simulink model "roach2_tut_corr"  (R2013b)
settings: Solver=VariableStepDiscrete  SolverMode=SingleTasking  StartTime=0.0  StopTime=100  RelTol=1e-3
undefined symbols (not defined in the file): add_latency, addr_width, Bit, bitfield, BitWidth, bram_latency, burst_size, casper_library_scopes, conv_latency, data_width, DelayLen, fan_latency, FFTSize, FFTStage, getfield, increment, led, Location, Lower, mult_latency, mux_latency, n_bits, n_bits_data, n_inputs, n_streams, n_taps, neg_latency, negate_latency, nsamples, pfb_size, pulse_len, reset_period, ROACH, ROACH2, snapshot, sx475t, sync_period, sync_period_bits, Upper, UseCounter, Width
libraries: xbsIndex_r4 x24444, casper_library_misc x73, xbsReplacements_r4 x34, casper_library_delays x14, xps_library x7
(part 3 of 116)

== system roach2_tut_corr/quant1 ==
  sync : Inport
  din : Inport  Port=2
  Constant : xbsIndex_r4/Constant  const=0  gui_display_data_type=Fixed-point  arith_type=Unsigned  n_bits=32  bin_pt=0  preci_type=Single  exp_width=8  frac_width=24  explicit_period=on  period=1  equ=P=C  opselect=C  inp2=PCIN>>17  opr=+  inp1=P  carry=CIN  dbl_ovrd=off  block_type=constant
  Constant1 : xbsIndex_r4/Constant  const=0  gui_display_data_type=Boolean  arith_type=Boolean  n_bits=32  bin_pt=0  preci_type=Single  exp_width=8  frac_width=24  explicit_period=on  period=1  equ=P=C  opselect=C  inp2=PCIN>>17  opr=+  inp1=P  carry=CIN  dbl_ovrd=off  block_type=constant
  Counter : xbsIndex_r4/Counter  cnt_type=Free Running  cnt_to=Inf  operation=Up  start_count=0  cnt_by_val=1  arith_type=Unsigned  n_bits=10  bin_pt=0  load_pin=off  rst=on  en=off  explicit_period=on  period=1  dbl_ovrd=off  use_behavioral_HDL=off  implementation=Fabric  block_type=counter
  Delay{1..3,5} (4 alike) : xbsIndex_r4/Delay  rst=off  infoeditControl=Selection of Reset will increase slice count due to use of real FFs and instead of SRLs  en=off  latency=1  dbl_ovrd=off  reg_retiming=on  block_type=delay
  Delay{6,18..19,25} (4 alike) : xbsIndex_r4/Delay  rst=off  infoeditControl=Selection of Reset will increase slice count due to use of real FFs and instead of SRLs  en=off  latency=1  dbl_ovrd=off  reg_retiming=off  block_type=delay
  Delay4 : xbsIndex_r4/Delay  rst=off  infoeditControl=Selection of Reset will increase slice count due to use of real FFs and instead of SRLs  en=off  latency=6  dbl_ovrd=off  reg_retiming=on  block_type=delay
  Logical5 : xbsIndex_r4/Logical  logical_function=OR  inputs=2  en=off  latency=0  precision=Full  arith_type=Unsigned  n_bits=8  bin_pt=2  align_bp=on  dbl_ovrd=off  block_type=logical
  Slice11 : xbsIndex_r4/Slice  nbits=16  boolean_output=off  mode=Lower Bit Location + Width  bit1=0  base1=MSB of Input  bit0=0  base0=LSB of Input  dbl_ovrd=off  block_type=slice
  Slice14 : xbsIndex_r4/Slice  nbits=16  boolean_output=off  mode=Lower Bit Location + Width  bit1=0  base1=MSB of Input  bit0=16  base0=LSB of Input  dbl_ovrd=off  block_type=slice
  bus_expand : Subsystem  AncestorBlock=casper_library_flow_control/bus_expand
  coeffs : Subsystem  Tag=xps:bram  AncestorBlock=xps_library/Shared_BRAM
  round0 : Subsystem
  round1 : Subsystem
  sync_out : Outport
  clip_out : Outport  Port=2
  dout0 : Outport  Port=3
  dout1 : Outport  Port=4
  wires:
  round0/2(clip) -> Logical5/1
  round1/2(clip) -> Logical5/2
  Delay19/1 -> Delay4/1
  coeffs/1(data_out) -> Delay1/1
  Slice14/1 -> round0/2(scale)
  Slice11/1 -> round1/2(scale)
  Delay18/1 -> Delay3/1
  Delay25/1 -> Delay2/1
  sync/1 -> Counter/1, Delay6/1
  Delay4/1 -> sync_out/1
  round0/1(dout) -> dout0/1
  Logical5/1 -> Delay5/1
  bus_expand/2(lsb_out1) -> Delay25/1
  round1/1(dout) -> dout1/1
  Delay1/1 -> Slice11/1, Slice14/1
  Delay2/1 -> round1/1(din)
  Delay3/1 -> round0/1(din)
  Delay5/1 -> clip_out/1
  bus_expand/1(msb_out2) -> Delay18/1
  din/1 -> bus_expand/1(bus_in)
  Delay6/1 -> Delay19/1
  Counter/1 -> coeffs/1(addr)
  Constant/1 -> coeffs/2(data_in)
  Constant1/1 -> coeffs/3(we)

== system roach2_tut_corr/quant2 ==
  sync : Inport
  din : Inport  Port=2
  Constant : xbsIndex_r4/Constant  const=0  gui_display_data_type=Fixed-point  arith_type=Unsigned  n_bits=32  bin_pt=0  preci_type=Single  exp_width=8  frac_width=24  explicit_period=on  period=1  equ=P=C  opselect=C  inp2=PCIN>>17  opr=+  inp1=P  carry=CIN  dbl_ovrd=off  block_type=constant
  Constant1 : xbsIndex_r4/Constant  const=0  gui_display_data_type=Boolean  arith_type=Boolean  n_bits=32  bin_pt=0  preci_type=Single  exp_width=8  frac_width=24  explicit_period=on  period=1  equ=P=C  opselect=C  inp2=PCIN>>17  opr=+  inp1=P  carry=CIN  dbl_ovrd=off  block_type=constant
  Counter : xbsIndex_r4/Counter  cnt_type=Free Running  cnt_to=Inf  operation=Up  start_count=0  cnt_by_val=1  arith_type=Unsigned  n_bits=10  bin_pt=0  load_pin=off  rst=on  en=off  explicit_period=on  period=1  dbl_ovrd=off  use_behavioral_HDL=off  implementation=Fabric  block_type=counter
  Delay{1..3,5} (4 alike) : xbsIndex_r4/Delay  rst=off  infoeditControl=Selection of Reset will increase slice count due to use of real FFs and instead of SRLs  en=off  latency=1  dbl_ovrd=off  reg_retiming=on  block_type=delay
  Delay{6,18..19,25} (4 alike) : xbsIndex_r4/Delay  rst=off  infoeditControl=Selection of Reset will increase slice count due to use of real FFs and instead of SRLs  en=off  latency=1  dbl_ovrd=off  reg_retiming=off  block_type=delay
  Delay4 : xbsIndex_r4/Delay  rst=off  infoeditControl=Selection of Reset will increase slice count due to use of real FFs and instead of SRLs  en=off  latency=6  dbl_ovrd=off  reg_retiming=on  block_type=delay
  Logical5 : xbsIndex_r4/Logical  logical_function=OR  inputs=2  en=off  latency=0  precision=Full  arith_type=Unsigned  n_bits=8  bin_pt=2  align_bp=on  dbl_ovrd=off  block_type=logical
  Slice11 : xbsIndex_r4/Slice  nbits=16  boolean_output=off  mode=Lower Bit Location + Width  bit1=0  base1=MSB of Input  bit0=0  base0=LSB of Input  dbl_ovrd=off  block_type=slice
  Slice14 : xbsIndex_r4/Slice  nbits=16  boolean_output=off  mode=Lower Bit Location + Width  bit1=0  base1=MSB of Input  bit0=16  base0=LSB of Input  dbl_ovrd=off  block_type=slice
  bus_expand : Subsystem  AncestorBlock=casper_library_flow_control/bus_expand
  coeffs : Subsystem  Tag=xps:bram  AncestorBlock=xps_library/Shared_BRAM
  round0 : Subsystem
  round1 : Subsystem
  sync_out : Outport
  clip_out : Outport  Port=2
  dout0 : Outport  Port=3
  dout1 : Outport  Port=4
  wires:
  round0/2(clip) -> Logical5/1
  round1/2(clip) -> Logical5/2
  Delay19/1 -> Delay4/1
  coeffs/1(data_out) -> Delay1/1
  Slice14/1 -> round0/2(scale)
  Slice11/1 -> round1/2(scale)
  Delay18/1 -> Delay3/1
  Delay25/1 -> Delay2/1
  sync/1 -> Counter/1, Delay6/1
  Delay4/1 -> sync_out/1
  round0/1(dout) -> dout0/1
  Logical5/1 -> Delay5/1
  bus_expand/2(lsb_out1) -> Delay25/1
  round1/1(dout) -> dout1/1
  Delay1/1 -> Slice11/1, Slice14/1
  Delay2/1 -> round1/1(din)
  Delay3/1 -> round0/1(din)
  Delay5/1 -> clip_out/1
  bus_expand/1(msb_out2) -> Delay18/1
  din/1 -> bus_expand/1(bus_in)
  Delay6/1 -> Delay19/1
  Counter/1 -> coeffs/1(addr)
  Constant/1 -> coeffs/2(data_in)
  Constant1/1 -> coeffs/3(we)

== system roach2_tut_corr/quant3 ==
  sync : Inport
  din : Inport  Port=2
  Constant : xbsIndex_r4/Constant  const=0  gui_display_data_type=Fixed-point  arith_type=Unsigned  n_bits=32  bin_pt=0  preci_type=Single  exp_width=8  frac_width=24  explicit_period=on  period=1  equ=P=C  opselect=C  inp2=PCIN>>17  opr=+  inp1=P  carry=CIN  dbl_ovrd=off  block_type=constant
  Constant1 : xbsIndex_r4/Constant  const=0  gui_display_data_type=Boolean  arith_type=Boolean  n_bits=32  bin_pt=0  preci_type=Single  exp_width=8  frac_width=24  explicit_period=on  period=1  equ=P=C  opselect=C  inp2=PCIN>>17  opr=+  inp1=P  carry=CIN  dbl_ovrd=off  block_type=constant
  Counter : xbsIndex_r4/Counter  cnt_type=Free Running  cnt_to=Inf  operation=Up  start_count=0  cnt_by_val=1  arith_type=Unsigned  n_bits=10  bin_pt=0  load_pin=off  rst=on  en=off  explicit_period=on  period=1  dbl_ovrd=off  use_behavioral_HDL=off  implementation=Fabric  block_type=counter
  Delay{1..3,5} (4 alike) : xbsIndex_r4/Delay  rst=off  infoeditControl=Selection of Reset will increase slice count due to use of real FFs and instead of SRLs  en=off  latency=1  dbl_ovrd=off  reg_retiming=on  block_type=delay
  Delay{6,18..19,25} (4 alike) : xbsIndex_r4/Delay  rst=off  infoeditControl=Selection of Reset will increase slice count due to use of real FFs and instead of SRLs  en=off  latency=1  dbl_ovrd=off  reg_retiming=off  block_type=delay
  Delay4 : xbsIndex_r4/Delay  rst=off  infoeditControl=Selection of Reset will increase slice count due to use of real FFs and instead of SRLs  en=off  latency=6  dbl_ovrd=off  reg_retiming=on  block_type=delay
  Logical5 : xbsIndex_r4/Logical  logical_function=OR  inputs=2  en=off  latency=0  precision=Full  arith_type=Unsigned  n_bits=8  bin_pt=2  align_bp=on  dbl_ovrd=off  block_type=logical
  Slice11 : xbsIndex_r4/Slice  nbits=16  boolean_output=off  mode=Lower Bit Location + Width  bit1=0  base1=MSB of Input  bit0=0  base0=LSB of Input  dbl_ovrd=off  block_type=slice
  Slice14 : xbsIndex_r4/Slice  nbits=16  boolean_output=off  mode=Lower Bit Location + Width  bit1=0  base1=MSB of Input  bit0=16  base0=LSB of Input  dbl_ovrd=off  block_type=slice
  bus_expand : Subsystem  AncestorBlock=casper_library_flow_control/bus_expand
  coeffs : Subsystem  Tag=xps:bram  AncestorBlock=xps_library/Shared_BRAM
  round0 : Subsystem
  round1 : Subsystem
  sync_out : Outport
  clip_out : Outport  Port=2
  dout0 : Outport  Port=3
  dout1 : Outport  Port=4
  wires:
  round0/2(clip) -> Logical5/1
  round1/2(clip) -> Logical5/2
  Delay19/1 -> Delay4/1
  coeffs/1(data_out) -> Delay1/1
  Slice14/1 -> round0/2(scale)
  Slice11/1 -> round1/2(scale)
  Delay18/1 -> Delay3/1
  Delay25/1 -> Delay2/1
  sync/1 -> Counter/1, Delay6/1
  Delay4/1 -> sync_out/1
  round0/1(dout) -> dout0/1
  Logical5/1 -> Delay5/1
  bus_expand/2(lsb_out1) -> Delay25/1
  round1/1(dout) -> dout1/1
  Delay1/1 -> Slice11/1, Slice14/1
  Delay2/1 -> round1/1(din)
  Delay3/1 -> round0/1(din)
  Delay5/1 -> clip_out/1
  bus_expand/1(msb_out2) -> Delay18/1
  din/1 -> bus_expand/1(bus_in)
  Delay6/1 -> Delay19/1
  Counter/1 -> coeffs/1(addr)
  Constant/1 -> coeffs/2(data_in)
  Constant1/1 -> coeffs/3(we)

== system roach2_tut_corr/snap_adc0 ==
  note: Generate stop when in circular capture mode
  note: Delay start of capture
  note: ctrl: bit0: Put a posedge here to enable a new capture. bit1: ignore external trigger and trigger immediately. bit2: ignore external write enable and capture on every FPGA clock. bit3: continuously capture data until we get an external stop command.
  note: Offset in vector from first element captured, used during circular capture
  note: Number of bytes in buffer and done bit
  note: Number of valid data samples to skip after trigger before starting capture
  note: Value on vin aligned with first sample on din captured
  din : Inport
  we : Inport  Port=2
  trig : Inport  Port=3
  add_del : xbsIndex_r4/Delay  rst=off  infoeditControl=Selection of Reset will increase slice count due to use of real FFs and instead of SRLs  en=off  latency=1  dbl_ovrd=off  reg_retiming=on  block_type=delay
  add_gen : Subsystem  AncestorBlock=casper_library_scopes/snapshot/add_gen
  basic_ctrl : Subsystem  AncestorBlock=casper_library_scopes/snapshot/basic_ctrl
  bram : Subsystem  Tag=xps:bram  AncestorBlock=xps_library/Shared_BRAM
  cast : xbsIndex_r4/Convert  gui_display_data_type=Fixed-point  arith_type=Unsigned  n_bits=32  bin_pt=0  float_type=Single  exp_bits=8  fraction_bits=24  quantization=Truncate  overflow=Wrap  en=off  latency=0  dbl_ovrd=off  pipeline=off  block_type=convert
  const0 : Constant  Value=0
  ctrl : Subsystem  Tag=xps:sw_reg  AncestorBlock=xps_library/software_register
  dat_del : xbsIndex_r4/Delay  rst=off  infoeditControl=Selection of Reset will increase slice count due to use of real FFs and instead of SRLs  en=off  latency=1  dbl_ovrd=off  reg_retiming=on  block_type=delay
  g_tr_en_cnt : Terminator
  gbram : Terminator
  gstatus : Terminator
  gval : Terminator
  never : xbsIndex_r4/Constant  const=0  gui_display_data_type=Fixed-point  arith_type=Boolean  n_bits=16  bin_pt=14  preci_type=Single  exp_width=8  frac_width=24  explicit_period=on  period=1  equ=P=C  opselect=C  inp2=PCIN>>17  opr=+  inp1=P  carry=CIN  dbl_ovrd=off  block_type=constant
  ri : xbsIndex_r4/Reinterpret  force_arith_type=on  arith_type=Unsigned  force_bin_pt=on  bin_pt=0  block_type=reinterpret
  status : Subsystem  Tag=xps:sw_reg  AncestorBlock=xps_library/software_register
  vin_const : xbsIndex_r4/Constant  const=0  gui_display_data_type=Fixed-point  arith_type=Boolean  n_bits=16  bin_pt=14  preci_type=Single  exp_width=8  frac_width=24  explicit_period=on  period=1  equ=P=C  opselect=C  inp2=PCIN>>17  opr=+  inp1=P  carry=CIN  dbl_ovrd=off  block_type=constant
  we_del : xbsIndex_r4/Delay  rst=off  infoeditControl=Selection of Reset will increase slice count due to use of real FFs and instead of SRLs  en=off  latency=1  dbl_ovrd=off  reg_retiming=on  block_type=delay
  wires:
  din/1 -> ri/1
  ri/1 -> cast/1
  cast/1 -> basic_ctrl/2(din)
  we/1 -> basic_ctrl/3(we)
  trig/1 -> basic_ctrl/4(trig)
  never/1 -> basic_ctrl/6(stopi)
  const0/1 -> ctrl/1(sim_1)
  ctrl/1(in_reg) -> basic_ctrl/5(ctrl)
  basic_ctrl/1(vout) -> add_gen/1(vin)
  basic_ctrl/2(dout) -> add_gen/2(din)
  basic_ctrl/3(we_o) -> add_gen/3(we)
  basic_ctrl/4(go) -> add_gen/4(go)
  basic_ctrl/5(stop) -> add_gen/5(cont)
  basic_ctrl/6(init) -> add_gen/6(init)
  add_gen/5(status) -> status/1(out_reg)
  status/1(sim_out) -> gstatus/1
  vin_const/1 -> basic_ctrl/1(vin)
  add_gen/1(vout) -> gval/1
  add_gen/6(en_cnt) -> g_tr_en_cnt/1
  add_gen/2(add) -> add_del/1
  add_gen/3(dout) -> dat_del/1
  add_gen/4(we_o) -> we_del/1
  add_del/1 -> bram/1(addr)
  dat_del/1 -> bram/2(data_in)
  we_del/1 -> bram/3(we)
  bram/1(data_out) -> gbram/1

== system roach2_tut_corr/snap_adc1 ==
  note: Generate stop when in circular capture mode
  note: Delay start of capture
  note: ctrl: bit0: Put a posedge here to enable a new capture. bit1: ignore external trigger and trigger immediately. bit2: ignore external write enable and capture on every FPGA clock. bit3: continuously capture data until we get an external stop command.
  note: Offset in vector from first element captured, used during circular capture
  note: Number of bytes in buffer and done bit
  note: Number of valid data samples to skip after trigger before starting capture
  note: Value on vin aligned with first sample on din captured
  din : Inport
  we : Inport  Port=2
  trig : Inport  Port=3
  add_del : xbsIndex_r4/Delay  rst=off  infoeditControl=Selection of Reset will increase slice count due to use of real FFs and instead of SRLs  en=off  latency=1  dbl_ovrd=off  reg_retiming=on  block_type=delay
  add_gen : Subsystem  AncestorBlock=casper_library_scopes/snapshot/add_gen
  basic_ctrl : Subsystem  AncestorBlock=casper_library_scopes/snapshot/basic_ctrl
  bram : Subsystem  Tag=xps:bram  AncestorBlock=xps_library/Shared_BRAM
  cast : xbsIndex_r4/Convert  gui_display_data_type=Fixed-point  arith_type=Unsigned  n_bits=32  bin_pt=0  float_type=Single  exp_bits=8  fraction_bits=24  quantization=Truncate  overflow=Wrap  en=off  latency=0  dbl_ovrd=off  pipeline=off  block_type=convert
  const0 : Constant  Value=0
  ctrl : Subsystem  Tag=xps:sw_reg  AncestorBlock=xps_library/software_register
  dat_del : xbsIndex_r4/Delay  rst=off  infoeditControl=Selection of Reset will increase slice count due to use of real FFs and instead of SRLs  en=off  latency=1  dbl_ovrd=off  reg_retiming=on  block_type=delay
  g_tr_en_cnt : Terminator
  gbram : Terminator
  gstatus : Terminator
  gval : Terminator
  never : xbsIndex_r4/Constant  const=0  gui_display_data_type=Fixed-point  arith_type=Boolean  n_bits=16  bin_pt=14  preci_type=Single  exp_width=8  frac_width=24  explicit_period=on  period=1  equ=P=C  opselect=C  inp2=PCIN>>17  opr=+  inp1=P  carry=CIN  dbl_ovrd=off  block_type=constant
  ri : xbsIndex_r4/Reinterpret  force_arith_type=on  arith_type=Unsigned  force_bin_pt=on  bin_pt=0  block_type=reinterpret
  status : Subsystem  Tag=xps:sw_reg  AncestorBlock=xps_library/software_register
  vin_const : xbsIndex_r4/Constant  const=0  gui_display_data_type=Fixed-point  arith_type=Boolean  n_bits=16  bin_pt=14  preci_type=Single  exp_width=8  frac_width=24  explicit_period=on  period=1  equ=P=C  opselect=C  inp2=PCIN>>17  opr=+  inp1=P  carry=CIN  dbl_ovrd=off  block_type=constant
  we_del : xbsIndex_r4/Delay  rst=off  infoeditControl=Selection of Reset will increase slice count due to use of real FFs and instead of SRLs  en=off  latency=1  dbl_ovrd=off  reg_retiming=on  block_type=delay
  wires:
  din/1 -> ri/1
  ri/1 -> cast/1
  cast/1 -> basic_ctrl/2(din)
  we/1 -> basic_ctrl/3(we)
  trig/1 -> basic_ctrl/4(trig)
  never/1 -> basic_ctrl/6(stopi)
  const0/1 -> ctrl/1(sim_1)
  ctrl/1(in_reg) -> basic_ctrl/5(ctrl)
  basic_ctrl/1(vout) -> add_gen/1(vin)
  basic_ctrl/2(dout) -> add_gen/2(din)
  basic_ctrl/3(we_o) -> add_gen/3(we)
  basic_ctrl/4(go) -> add_gen/4(go)
  basic_ctrl/5(stop) -> add_gen/5(cont)
  basic_ctrl/6(init) -> add_gen/6(init)
  add_gen/5(status) -> status/1(out_reg)
  status/1(sim_out) -> gstatus/1
  vin_const/1 -> basic_ctrl/1(vin)
  add_gen/1(vout) -> gval/1
  add_gen/6(en_cnt) -> g_tr_en_cnt/1
  add_gen/2(add) -> add_del/1
  add_gen/3(dout) -> dat_del/1
  add_gen/4(we_o) -> we_del/1
  add_del/1 -> bram/1(addr)
  dat_del/1 -> bram/2(data_in)
  we_del/1 -> bram/3(we)
  bram/1(data_out) -> gbram/1

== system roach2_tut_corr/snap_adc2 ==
  note: Generate stop when in circular capture mode
  note: Delay start of capture
  note: ctrl: bit0: Put a posedge here to enable a new capture. bit1: ignore external trigger and trigger immediately. bit2: ignore external write enable and capture on every FPGA clock. bit3: continuously capture data until we get an external stop command.
  note: Offset in vector from first element captured, used during circular capture
  note: Number of bytes in buffer and done bit
  note: Number of valid data samples to skip after trigger before starting capture
  note: Value on vin aligned with first sample on din captured
  din : Inport
  we : Inport  Port=2
  trig : Inport  Port=3
  add_del : xbsIndex_r4/Delay  rst=off  infoeditControl=Selection of Reset will increase slice count due to use of real FFs and instead of SRLs  en=off  latency=1  dbl_ovrd=off  reg_retiming=on  block_type=delay
  add_gen : Subsystem  AncestorBlock=casper_library_scopes/snapshot/add_gen
  basic_ctrl : Subsystem  AncestorBlock=casper_library_scopes/snapshot/basic_ctrl
  bram : Subsystem  Tag=xps:bram  AncestorBlock=xps_library/Shared_BRAM
  cast : xbsIndex_r4/Convert  gui_display_data_type=Fixed-point  arith_type=Unsigned  n_bits=32  bin_pt=0  float_type=Single  exp_bits=8  fraction_bits=24  quantization=Truncate  overflow=Wrap  en=off  latency=0  dbl_ovrd=off  pipeline=off  block_type=convert
  const0 : Constant  Value=0
  ctrl : Subsystem  Tag=xps:sw_reg  AncestorBlock=xps_library/software_register
  dat_del : xbsIndex_r4/Delay  rst=off  infoeditControl=Selection of Reset will increase slice count due to use of real FFs and instead of SRLs  en=off  latency=1  dbl_ovrd=off  reg_retiming=on  block_type=delay
  g_tr_en_cnt : Terminator
  gbram : Terminator
  gstatus : Terminator
  gval : Terminator
  never : xbsIndex_r4/Constant  const=0  gui_display_data_type=Fixed-point  arith_type=Boolean  n_bits=16  bin_pt=14  preci_type=Single  exp_width=8  frac_width=24  explicit_period=on  period=1  equ=P=C  opselect=C  inp2=PCIN>>17  opr=+  inp1=P  carry=CIN  dbl_ovrd=off  block_type=constant
  ri : xbsIndex_r4/Reinterpret  force_arith_type=on  arith_type=Unsigned  force_bin_pt=on  bin_pt=0  block_type=reinterpret
  status : Subsystem  Tag=xps:sw_reg  AncestorBlock=xps_library/software_register
  vin_const : xbsIndex_r4/Constant  const=0  gui_display_data_type=Fixed-point  arith_type=Boolean  n_bits=16  bin_pt=14  preci_type=Single  exp_width=8  frac_width=24  explicit_period=on  period=1  equ=P=C  opselect=C  inp2=PCIN>>17  opr=+  inp1=P  carry=CIN  dbl_ovrd=off  block_type=constant
  we_del : xbsIndex_r4/Delay  rst=off  infoeditControl=Selection of Reset will increase slice count due to use of real FFs and instead of SRLs  en=off  latency=1  dbl_ovrd=off  reg_retiming=on  block_type=delay
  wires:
  din/1 -> ri/1
  ri/1 -> cast/1
  cast/1 -> basic_ctrl/2(din)
  we/1 -> basic_ctrl/3(we)
  trig/1 -> basic_ctrl/4(trig)
  never/1 -> basic_ctrl/6(stopi)
  const0/1 -> ctrl/1(sim_1)
  ctrl/1(in_reg) -> basic_ctrl/5(ctrl)
  basic_ctrl/1(vout) -> add_gen/1(vin)
  basic_ctrl/2(dout) -> add_gen/2(din)
  basic_ctrl/3(we_o) -> add_gen/3(we)
  basic_ctrl/4(go) -> add_gen/4(go)
  basic_ctrl/5(stop) -> add_gen/5(cont)
  basic_ctrl/6(init) -> add_gen/6(init)
  add_gen/5(status) -> status/1(out_reg)
  status/1(sim_out) -> gstatus/1
  vin_const/1 -> basic_ctrl/1(vin)
  add_gen/1(vout) -> gval/1
  add_gen/6(en_cnt) -> g_tr_en_cnt/1
  add_gen/2(add) -> add_del/1
  add_gen/3(dout) -> dat_del/1
  add_gen/4(we_o) -> we_del/1
  add_del/1 -> bram/1(addr)
  dat_del/1 -> bram/2(data_in)
  we_del/1 -> bram/3(we)
  bram/1(data_out) -> gbram/1

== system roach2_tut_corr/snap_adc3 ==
  note: Generate stop when in circular capture mode
  note: Delay start of capture
  note: ctrl: bit0: Put a posedge here to enable a new capture. bit1: ignore external trigger and trigger immediately. bit2: ignore external write enable and capture on every FPGA clock. bit3: continuously capture data until we get an external stop command.
  note: Offset in vector from first element captured, used during circular capture
  note: Number of bytes in buffer and done bit
  note: Number of valid data samples to skip after trigger before starting capture
  note: Value on vin aligned with first sample on din captured
  din : Inport
  we : Inport  Port=2
  trig : Inport  Port=3
  add_del : xbsIndex_r4/Delay  rst=off  infoeditControl=Selection of Reset will increase slice count due to use of real FFs and instead of SRLs  en=off  latency=1  dbl_ovrd=off  reg_retiming=on  block_type=delay
  add_gen : Subsystem  AncestorBlock=casper_library_scopes/snapshot/add_gen
  basic_ctrl : Subsystem  AncestorBlock=casper_library_scopes/snapshot/basic_ctrl
  bram : Subsystem  Tag=xps:bram  AncestorBlock=xps_library/Shared_BRAM
  cast : xbsIndex_r4/Convert  gui_display_data_type=Fixed-point  arith_type=Unsigned  n_bits=32  bin_pt=0  float_type=Single  exp_bits=8  fraction_bits=24  quantization=Truncate  overflow=Wrap  en=off  latency=0  dbl_ovrd=off  pipeline=off  block_type=convert
  const0 : Constant  Value=0
  ctrl : Subsystem  Tag=xps:sw_reg  AncestorBlock=xps_library/software_register
  dat_del : xbsIndex_r4/Delay  rst=off  infoeditControl=Selection of Reset will increase slice count due to use of real FFs and instead of SRLs  en=off  latency=1  dbl_ovrd=off  reg_retiming=on  block_type=delay
  g_tr_en_cnt : Terminator
  gbram : Terminator
  gstatus : Terminator
  gval : Terminator
  never : xbsIndex_r4/Constant  const=0  gui_display_data_type=Fixed-point  arith_type=Boolean  n_bits=16  bin_pt=14  preci_type=Single  exp_width=8  frac_width=24  explicit_period=on  period=1  equ=P=C  opselect=C  inp2=PCIN>>17  opr=+  inp1=P  carry=CIN  dbl_ovrd=off  block_type=constant
  ri : xbsIndex_r4/Reinterpret  force_arith_type=on  arith_type=Unsigned  force_bin_pt=on  bin_pt=0  block_type=reinterpret
  status : Subsystem  Tag=xps:sw_reg  AncestorBlock=xps_library/software_register
  vin_const : xbsIndex_r4/Constant  const=0  gui_display_data_type=Fixed-point  arith_type=Boolean  n_bits=16  bin_pt=14  preci_type=Single  exp_width=8  frac_width=24  explicit_period=on  period=1  equ=P=C  opselect=C  inp2=PCIN>>17  opr=+  inp1=P  carry=CIN  dbl_ovrd=off  block_type=constant
  we_del : xbsIndex_r4/Delay  rst=off  infoeditControl=Selection of Reset will increase slice count due to use of real FFs and instead of SRLs  en=off  latency=1  dbl_ovrd=off  reg_retiming=on  block_type=delay
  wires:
  din/1 -> ri/1
  ri/1 -> cast/1
  cast/1 -> basic_ctrl/2(din)
  we/1 -> basic_ctrl/3(we)
  trig/1 -> basic_ctrl/4(trig)
  never/1 -> basic_ctrl/6(stopi)
  const0/1 -> ctrl/1(sim_1)
  ctrl/1(in_reg) -> basic_ctrl/5(ctrl)
  basic_ctrl/1(vout) -> add_gen/1(vin)
  basic_ctrl/2(dout) -> add_gen/2(din)
  basic_ctrl/3(we_o) -> add_gen/3(we)
  basic_ctrl/4(go) -> add_gen/4(go)
  basic_ctrl/5(stop) -> add_gen/5(cont)
  basic_ctrl/6(init) -> add_gen/6(init)
  add_gen/5(status) -> status/1(out_reg)
  status/1(sim_out) -> gstatus/1
  vin_const/1 -> basic_ctrl/1(vin)
  add_gen/1(vout) -> gval/1
  add_gen/6(en_cnt) -> g_tr_en_cnt/1
  add_gen/2(add) -> add_del/1
  add_gen/3(dout) -> dat_del/1
  add_gen/4(we_o) -> we_del/1
  add_del/1 -> bram/1(addr)
  dat_del/1 -> bram/2(data_in)
  we_del/1 -> bram/3(we)
  bram/1(data_out) -> gbram/1

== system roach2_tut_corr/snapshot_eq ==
  in_quant0 : Inport
  in_quant1 : Inport  Port=2
  in_quant2 : Inport  Port=3
  in_quant3 : Inport  Port=4
  we : Inport  Port=5
  trig : Inport  Port=6
  assert_quant{0..3} (4 alike) : xbsIndex_r4/Assert  assert_type=on  type_source=Explicitly  gui_display_data_type=Fixed-point  arith_type=Unsigned  n_bits=16  bin_pt=0  preci_type=Single  exp_width=8  frac_width=24  assert_rate=off  rate_source=Explicitly  period=1  output_port=on  block_type=assert
  buscreate : Subsystem  AncestorBlock=casper_library_flow_control/bus_create
  ss : Subsystem  Tag=casper:snapshot  AncestorBlock=casper_library_scopes/snapshot
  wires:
  buscreate/1(bus_out) -> ss/1(din)
  in_quant0/1 -> assert_quant0/1
  assert_quant0/1 -> buscreate/1(in1)
  in_quant1/1 -> assert_quant1/1
  assert_quant1/1 -> buscreate/2(in2)
  in_quant2/1 -> assert_quant2/1
  assert_quant2/1 -> buscreate/3(in3)
  in_quant3/1 -> assert_quant3/1
  assert_quant3/1 -> buscreate/4(in4)
  we/1 -> ss/2(we)
  trig/1 -> ss/3(trig)

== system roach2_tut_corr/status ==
  out_reg : Inport
  assert_reg : xbsIndex_r4/Assert  assert_type=on  type_source=Explicitly  gui_display_data_type=Fixed-point  arith_type=Unsigned  n_bits=32  bin_pt=0  preci_type=Single  exp_width=8  frac_width=24  assert_rate=off  rate_source=Explicitly  period=1  output_port=on  block_type=assert
  cast_gw : xbsIndex_r4/Convert  gui_display_data_type=Fixed-point  arith_type=Unsigned  n_bits=32  bin_pt=0  float_type=Single  exp_bits=8  fraction_bits=24  quantization=Truncate  overflow=Wrap  en=off  latency=0  dbl_ovrd=off  pipeline=off  block_type=convert
  io_delay : xbsIndex_r4/Delay  rst=off  infoeditControl=Selection of Reset will increase slice count due to use of real FFs and instead of SRLs  en=off  latency=0  dbl_ovrd=off  reg_retiming=on  block_type=delay
  reint1 : xbsIndex_r4/Reinterpret  force_arith_type=on  arith_type=Unsigned  force_bin_pt=on  bin_pt=0  block_type=reinterpret
  roach2_tut_corr_status_user_data_in : xbsIndex_r4/Gateway Out  inherit_from_input=off  hdl_port=on  timing_constraint=None  locs_specified=off  LOCs={}  UseAsDAC=off  DACChannel='1'  block_type=gatewayout
  sim_out : Outport
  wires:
  io_delay/1 -> cast_gw/1
  cast_gw/1 -> roach2_tut_corr_status_user_data_in/1
  roach2_tut_corr_status_user_data_in/1 -> sim_out/1
  out_reg/1 -> assert_reg/1
  assert_reg/1 -> reint1/1
  reint1/1 -> io_delay/1

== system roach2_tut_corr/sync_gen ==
  arm : Inport
  pps : Inport  Port=2
  Constant : xbsIndex_r4/Constant  const=sync_period  gui_display_data_type=Fixed-point  arith_type=Unsigned  n_bits=sync_period_bits+1  bin_pt=0  preci_type=Single  exp_width=8  frac_width=24  explicit_period=on  period=1  equ=P=C  opselect=C  inp2=PCIN>>17  opr=+  inp1=P  carry=CIN  dbl_ovrd=off  block_type=constant
  Delay1 : xbsIndex_r4/Delay  rst=off  infoeditControl=Selection of Reset will increase slice count due to use of real FFs and instead of SRLs  en=off  latency=1  dbl_ovrd=off  reg_retiming=on  block_type=delay
  Delay2 : xbsIndex_r4/Delay  rst=off  infoeditControl=Selection of Reset will increase slice count due to use of real FFs and instead of SRLs  en=off  latency=1  dbl_ovrd=off  reg_retiming=on  block_type=delay
  rst_gen : Subsystem
  sync_gen : Subsystem
  mrst : Outport
  sync : Outport  Port=2
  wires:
  arm/1 -> rst_gen/1(arm)
  pps/1 -> rst_gen/2(sync_in)
  sync_gen/1(sync) -> Delay2/1
  rst_gen/1(mrst) -> sync_gen/1(rst), Delay1/1
  Delay1/1 -> mrst/1
  Delay2/1 -> sync/1
  Constant/1 -> sync_gen/2(sync_period)

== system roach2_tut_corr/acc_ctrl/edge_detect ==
  in : Inport
  Delay : xbsIndex_r4/Delay  rst=off  infoeditControl=Selection of Reset will increase slice count due to use of real FFs and instead of SRLs  en=off  latency=1  dbl_ovrd=off  reg_retiming=on  block_type=delay
  Inverter : xbsIndex_r4/Inverter  en=off  latency=0  dbl_ovrd=off  block_type=inv
  edge_op : xbsIndex_r4/Logical  logical_function=NOR  inputs=2  en=off  latency=0  precision=Full  arith_type=Unsigned  n_bits=8  bin_pt=2  align_bp=on  dbl_ovrd=off  block_type=logical
  out : Outport
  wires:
  Inverter/1 -> edge_op/1
  edge_op/1 -> out/1
  in/1 -> Inverter/1, Delay/1
  Delay/1 -> edge_op/2

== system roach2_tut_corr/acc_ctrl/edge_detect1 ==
  in : Inport
  Delay : xbsIndex_r4/Delay  rst=off  infoeditControl=Selection of Reset will increase slice count due to use of real FFs and instead of SRLs  en=off  latency=1  dbl_ovrd=off  reg_retiming=on  block_type=delay
  Inverter : xbsIndex_r4/Inverter  en=off  latency=0  dbl_ovrd=off  block_type=inv
  edge_op : xbsIndex_r4/Logical  logical_function=NOR  inputs=2  en=off  latency=0  precision=Full  arith_type=Unsigned  n_bits=8  bin_pt=2  align_bp=on  dbl_ovrd=off  block_type=logical
  out : Outport
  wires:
  Inverter/1 -> edge_op/1
  edge_op/1 -> out/1
  in/1 -> Inverter/1, Delay/1
  Delay/1 -> edge_op/2

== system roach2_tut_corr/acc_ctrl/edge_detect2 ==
  in : Inport
  Delay : xbsIndex_r4/Delay  rst=off  infoeditControl=Selection of Reset will increase slice count due to use of real FFs and instead of SRLs  en=off  latency=1  dbl_ovrd=off  reg_retiming=on  block_type=delay
  Inverter : xbsIndex_r4/Inverter  en=off  latency=0  dbl_ovrd=off  block_type=inv
  edge_op : xbsIndex_r4/Logical  logical_function=NOR  inputs=2  en=off  latency=0  precision=Full  arith_type=Unsigned  n_bits=8  bin_pt=2  align_bp=on  dbl_ovrd=off  block_type=logical
  out : Outport
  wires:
  Inverter/1 -> edge_op/1
  edge_op/1 -> out/1
  in/1 -> Inverter/1, Delay/1
  Delay/1 -> edge_op/2

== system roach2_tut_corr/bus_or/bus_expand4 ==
  bus_in : Inport
  slice1 : xbsIndex_r4/Slice  nbits=1  boolean_output=on  mode=Upper Bit Location + Width  bit1=-3  base1=MSB of Input  bit0=0  base0=LSB of Input  dbl_ovrd=off  block_type=slice
  slice2 : xbsIndex_r4/Slice  nbits=1  boolean_output=on  mode=Upper Bit Location + Width  bit1=-2  base1=MSB of Input  bit0=0  base0=LSB of Input  dbl_ovrd=off  block_type=slice
  slice3 : xbsIndex_r4/Slice  nbits=1  boolean_output=on  mode=Upper Bit Location + Width  bit1=-1  base1=MSB of Input  bit0=0  base0=LSB of Input  dbl_ovrd=off  block_type=slice
  slice4 : xbsIndex_r4/Slice  nbits=1  boolean_output=on  mode=Upper Bit Location + Width  bit1=0  base1=MSB of Input  bit0=0  base0=LSB of Input  dbl_ovrd=off  block_type=slice
  msb_out4 : Outport
  out3 : Outport  Port=2
  out2 : Outport  Port=3
  lsb_out1 : Outport  Port=4
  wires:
  bus_in/1 -> slice4/1, slice3/1, slice2/1, slice1/1
  slice4/1 -> msb_out4/1
  slice3/1 -> out3/1
  slice2/1 -> out2/1
  slice1/1 -> lsb_out1/1

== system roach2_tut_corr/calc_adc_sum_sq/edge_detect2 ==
  in : Inport
  Delay : xbsIndex_r4/Delay  rst=off  infoeditControl=Selection of Reset will increase slice count due to use of real FFs and instead of SRLs  en=off  latency=1  dbl_ovrd=off  reg_retiming=on  block_type=delay
  Inverter : xbsIndex_r4/Inverter  en=off  latency=0  dbl_ovrd=off  block_type=inv
  edge_op : xbsIndex_r4/Logical  logical_function=AND  inputs=2  en=off  latency=0  precision=Full  arith_type=Unsigned  n_bits=8  bin_pt=2  align_bp=on  dbl_ovrd=off  block_type=logical
  out : Outport
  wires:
  Inverter/1 -> edge_op/1
  edge_op/1 -> out/1
  in/1 -> Inverter/1, Delay/1
  Delay/1 -> edge_op/2

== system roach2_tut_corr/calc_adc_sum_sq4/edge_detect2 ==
  in : Inport
  Delay : xbsIndex_r4/Delay  rst=off  infoeditControl=Selection of Reset will increase slice count due to use of real FFs and instead of SRLs  en=off  latency=1  dbl_ovrd=off  reg_retiming=on  block_type=delay
  Inverter : xbsIndex_r4/Inverter  en=off  latency=0  dbl_ovrd=off  block_type=inv
  edge_op : xbsIndex_r4/Logical  logical_function=AND  inputs=2  en=off  latency=0  precision=Full  arith_type=Unsigned  n_bits=8  bin_pt=2  align_bp=on  dbl_ovrd=off  block_type=logical
  out : Outport
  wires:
  Inverter/1 -> edge_op/1
  edge_op/1 -> out/1
  in/1 -> Inverter/1, Delay/1
  Delay/1 -> edge_op/2

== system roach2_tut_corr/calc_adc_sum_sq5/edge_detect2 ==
  in : Inport
  Delay : xbsIndex_r4/Delay  rst=off  infoeditControl=Selection of Reset will increase slice count due to use of real FFs and instead of SRLs  en=off  latency=1  dbl_ovrd=off  reg_retiming=on  block_type=delay
  Inverter : xbsIndex_r4/Inverter  en=off  latency=0  dbl_ovrd=off  block_type=inv
  edge_op : xbsIndex_r4/Logical  logical_function=AND  inputs=2  en=off  latency=0  precision=Full  arith_type=Unsigned  n_bits=8  bin_pt=2  align_bp=on  dbl_ovrd=off  block_type=logical
  out : Outport
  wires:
  Inverter/1 -> edge_op/1
  edge_op/1 -> out/1
  in/1 -> Inverter/1, Delay/1
  Delay/1 -> edge_op/2

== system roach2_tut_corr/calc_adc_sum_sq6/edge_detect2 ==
  in : Inport
  Delay : xbsIndex_r4/Delay  rst=off  infoeditControl=Selection of Reset will increase slice count due to use of real FFs and instead of SRLs  en=off  latency=1  dbl_ovrd=off  reg_retiming=on  block_type=delay
  Inverter : xbsIndex_r4/Inverter  en=off  latency=0  dbl_ovrd=off  block_type=inv
  edge_op : xbsIndex_r4/Logical  logical_function=AND  inputs=2  en=off  latency=0  precision=Full  arith_type=Unsigned  n_bits=8  bin_pt=2  align_bp=on  dbl_ovrd=off  block_type=logical
  out : Outport
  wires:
  Inverter/1 -> edge_op/1
  edge_op/1 -> out/1
  in/1 -> Inverter/1, Delay/1
  Delay/1 -> edge_op/2

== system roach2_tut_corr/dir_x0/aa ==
  a+bi : Inport
  c+di : Inport  Port=2
  new_acc : Inport  Port=3
  Counter : xbsIndex_r4/Counter  cnt_type=Free Running  cnt_to=Inf  operation=Up  start_count=0  cnt_by_val=1  arith_type=Unsigned  n_bits=chan_bits  bin_pt=0  load_pin=off  rst=on  en=on  explicit_period=off  period=1  dbl_ovrd=off  use_behavioral_HDL=off  implementation=Fabric  use_rpm=on  block_type=counter
  Delay3 : xbsIndex_r4/Delay  rst=off  infoeditControl=Selection of Reset will increase slice count due to use of real FFs and instead of SRLs  en=off  latency=4  dbl_ovrd=off  reg_retiming=off  block_type=delay
  Gateway Out{,1..3} (4 alike) : xbsIndex_r4/Gateway Out  inherit_from_input=off  hdl_port=on  timing_constraint=None  locs_specified=off  LOCs={}  UseAsDAC=off  DACChannel='1'  block_type=gatewayout
  Reinterpret : xbsIndex_r4/Reinterpret  force_arith_type=on  arith_type=Unsigned  force_bin_pt=on  bin_pt=0  block_type=reinterpret
  Scope : Scope  NumInputPorts=4
  Terminator : Terminator
  c_to_ri : Subsystem
  c_to_ri1 : Subsystem
  cmult_dsp48e : Subsystem  AncestorBlock=casper_library_multipliers/cmult_dsp48e
  real : Subsystem  Tag=xps:bram  AncestorBlock=xps_library/Shared_BRAM
  vacc_32bit : Subsystem
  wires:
  Reinterpret/1 -> real/2(data_in), Gateway Out1/1
  Counter/1 -> real/1(addr), Gateway Out/1
  vacc_32bit/2(valid) -> Counter/2, real/3(we), Gateway Out2/1
  Delay3/1 -> Counter/1, vacc_32bit/2(new_acc), Gateway Out3/1
  c+di/1 -> c_to_ri1/1(c)
  a+bi/1 -> c_to_ri/1(c)
  c_to_ri1/2(im) -> cmult_dsp48e/4(b_im)
  c_to_ri1/1(re) -> cmult_dsp48e/3(b_re)
  c_to_ri/2(im) -> cmult_dsp48e/2(a_im)
  c_to_ri/1(re) -> cmult_dsp48e/1(a_re)
  vacc_32bit/1(dout) -> Reinterpret/1
  new_acc/1 -> Delay3/1
  cmult_dsp48e/1(c_re) -> vacc_32bit/1(din)
  real/1(data_out) -> Terminator/1
  Gateway Out/1 -> Scope/1
  Gateway Out1/1 -> Scope/2
  Gateway Out2/1 -> Scope/3
  Gateway Out3/1 -> Scope/4

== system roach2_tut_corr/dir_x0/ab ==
  a+bi : Inport
  c+di : Inport  Port=2
  new_acc : Inport  Port=3
  Counter : xbsIndex_r4/Counter  cnt_type=Free Running  cnt_to=Inf  operation=Up  start_count=0  cnt_by_val=1  arith_type=Unsigned  n_bits=11  bin_pt=0  load_pin=off  rst=on  en=on  explicit_period=off  period=1  dbl_ovrd=off  use_behavioral_HDL=off  implementation=Fabric  use_rpm=on  block_type=counter
  Delay3 : xbsIndex_r4/Delay  rst=off  infoeditControl=Selection of Reset will increase slice count due to use of real FFs and instead of SRLs  en=off  latency=4  dbl_ovrd=off  reg_retiming=off  block_type=delay
  Reinterpret : xbsIndex_r4/Reinterpret  force_arith_type=on  arith_type=Unsigned  force_bin_pt=on  bin_pt=0  block_type=reinterpret
  Reinterpret1 : xbsIndex_r4/Reinterpret  force_arith_type=on  arith_type=Unsigned  force_bin_pt=on  bin_pt=0  block_type=reinterpret
  c_to_ri : Subsystem
  c_to_ri1 : Subsystem
  cmult_dsp48e : Subsystem  AncestorBlock=casper_library_multipliers/cmult_dsp48e
  imag : Subsystem  Tag=xps:bram  AncestorBlock=xps_library/Shared_BRAM
  real : Subsystem  Tag=xps:bram  AncestorBlock=xps_library/Shared_BRAM
  vacc_0 : Subsystem
  vacc_1 : Subsystem
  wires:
  Counter/1 -> real/1(addr), imag/1(addr)
  vacc_1/1(dout) -> Reinterpret1/1
  Reinterpret1/1 -> imag/2(data_in)
  vacc_1/2(valid) -> imag/3(we)
  Reinterpret/1 -> real/2(data_in)
  vacc_0/2(valid) -> real/3(we), Counter/2
  vacc_0/1(dout) -> Reinterpret/1
  new_acc/1 -> Delay3/1
  Delay3/1 -> vacc_0/2(new_acc), Counter/1, vacc_1/2(new_acc)
  c+di/1 -> c_to_ri1/1(c)
  a+bi/1 -> c_to_ri/1(c)
  c_to_ri1/2(im) -> cmult_dsp48e/4(b_im)
  c_to_ri1/1(re) -> cmult_dsp48e/3(b_re)
  c_to_ri/2(im) -> cmult_dsp48e/2(a_im)
  c_to_ri/1(re) -> cmult_dsp48e/1(a_re)
  cmult_dsp48e/2(c_im) -> vacc_1/1(din)
  cmult_dsp48e/1(c_re) -> vacc_0/1(din)

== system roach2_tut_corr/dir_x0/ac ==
  a+bi : Inport
  c+di : Inport  Port=2
  new_acc : Inport  Port=3
  Counter : xbsIndex_r4/Counter  cnt_type=Free Running  cnt_to=Inf  operation=Up  start_count=0  cnt_by_val=1  arith_type=Unsigned  n_bits=11  bin_pt=0  load_pin=off  rst=on  en=on  explicit_period=off  period=1  dbl_ovrd=off  use_behavioral_HDL=off  implementation=Fabric  use_rpm=on  block_type=counter
  Delay3 : xbsIndex_r4/Delay  rst=off  infoeditControl=Selection of Reset will increase slice count due to use of real FFs and instead of SRLs  en=off  latency=4  dbl_ovrd=off  reg_retiming=off  block_type=delay
  Reinterpret : xbsIndex_r4/Reinterpret  force_arith_type=on  arith_type=Unsigned  force_bin_pt=on  bin_pt=0  block_type=reinterpret
  Reinterpret1 : xbsIndex_r4/Reinterpret  force_arith_type=on  arith_type=Unsigned  force_bin_pt=on  bin_pt=0  block_type=reinterpret
  c_to_ri : Subsystem
  c_to_ri1 : Subsystem
  cmult_dsp48e : Subsystem  AncestorBlock=casper_library_multipliers/cmult_dsp48e
  imag : Subsystem  Tag=xps:bram  AncestorBlock=xps_library/Shared_BRAM
  real : Subsystem  Tag=xps:bram  AncestorBlock=xps_library/Shared_BRAM
  vacc_0 : Subsystem
  vacc_1 : Subsystem
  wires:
  cmult_dsp48e/1(c_re) -> vacc_0/1(din)
  cmult_dsp48e/2(c_im) -> vacc_1/1(din)
  c_to_ri/1(re) -> cmult_dsp48e/1(a_re)
  c_to_ri/2(im) -> cmult_dsp48e/2(a_im)
  c_to_ri1/1(re) -> cmult_dsp48e/3(b_re)
  c_to_ri1/2(im) -> cmult_dsp48e/4(b_im)
  a+bi/1 -> c_to_ri/1(c)
  c+di/1 -> c_to_ri1/1(c)
  Delay3/1 -> vacc_1/2(new_acc), Counter/1, vacc_0/2(new_acc)
  new_acc/1 -> Delay3/1
  vacc_0/1(dout) -> Reinterpret/1
  vacc_0/2(valid) -> Counter/2, real/3(we)
  Reinterpret/1 -> real/2(data_in)
  vacc_1/2(valid) -> imag/3(we)
  Reinterpret1/1 -> imag/2(data_in)
  vacc_1/1(dout) -> Reinterpret1/1
  Counter/1 -> imag/1(addr), real/1(addr)

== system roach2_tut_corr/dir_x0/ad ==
  a+bi : Inport
  c+di : Inport  Port=2
  new_acc : Inport  Port=3
  Counter : xbsIndex_r4/Counter  cnt_type=Free Running  cnt_to=Inf  operation=Up  start_count=0  cnt_by_val=1  arith_type=Unsigned  n_bits=11  bin_pt=0  load_pin=off  rst=on  en=on  explicit_period=off  period=1  dbl_ovrd=off  use_behavioral_HDL=off  implementation=Fabric  use_rpm=on  block_type=counter
  Delay3 : xbsIndex_r4/Delay  rst=off  infoeditControl=Selection of Reset will increase slice count due to use of real FFs and instead of SRLs  en=off  latency=4  dbl_ovrd=off  reg_retiming=off  block_type=delay
  Reinterpret : xbsIndex_r4/Reinterpret  force_arith_type=on  arith_type=Unsigned  force_bin_pt=on  bin_pt=0  block_type=reinterpret
  Reinterpret1 : xbsIndex_r4/Reinterpret  force_arith_type=on  arith_type=Unsigned  force_bin_pt=on  bin_pt=0  block_type=reinterpret
  c_to_ri : Subsystem
  c_to_ri1 : Subsystem
  cmult_dsp48e : Subsystem  AncestorBlock=casper_library_multipliers/cmult_dsp48e
  imag : Subsystem  Tag=xps:bram  AncestorBlock=xps_library/Shared_BRAM
  real : Subsystem  Tag=xps:bram  AncestorBlock=xps_library/Shared_BRAM
  vacc_0 : Subsystem
  vacc_1 : Subsystem
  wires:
  Counter/1 -> real/1(addr), imag/1(addr)
  vacc_1/1(dout) -> Reinterpret1/1
  Reinterpret1/1 -> imag/2(data_in)
  vacc_1/2(valid) -> imag/3(we)
  Reinterpret/1 -> real/2(data_in)
  vacc_0/2(valid) -> real/3(we), Counter/2
  vacc_0/1(dout) -> Reinterpret/1
  new_acc/1 -> Delay3/1
  Delay3/1 -> vacc_0/2(new_acc), Counter/1, vacc_1/2(new_acc)
  c+di/1 -> c_to_ri1/1(c)
  a+bi/1 -> c_to_ri/1(c)
  c_to_ri1/2(im) -> cmult_dsp48e/4(b_im)
  c_to_ri1/1(re) -> cmult_dsp48e/3(b_re)
  c_to_ri/2(im) -> cmult_dsp48e/2(a_im)
  c_to_ri/1(re) -> cmult_dsp48e/1(a_re)
  cmult_dsp48e/2(c_im) -> vacc_1/1(din)
  cmult_dsp48e/1(c_re) -> vacc_0/1(din)

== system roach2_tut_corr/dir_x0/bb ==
  a+bi : Inport
  c+di : Inport  Port=2
  new_acc : Inport  Port=3
  Counter : xbsIndex_r4/Counter  cnt_type=Free Running  cnt_to=Inf  operation=Up  start_count=0  cnt_by_val=1  arith_type=Unsigned  n_bits=chan_bits  bin_pt=0  load_pin=off  rst=on  en=on  explicit_period=off  period=1  dbl_ovrd=off  use_behavioral_HDL=off  implementation=Fabric  use_rpm=on  block_type=counter
  Delay3 : xbsIndex_r4/Delay  rst=off  infoeditControl=Selection of Reset will increase slice count due to use of real FFs and instead of SRLs  en=off  latency=4  dbl_ovrd=off  reg_retiming=off  block_type=delay
  Gateway Out{,1..3} (4 alike) : xbsIndex_r4/Gateway Out  inherit_from_input=off  hdl_port=on  timing_constraint=None  locs_specified=off  LOCs={}  UseAsDAC=off  DACChannel='1'  block_type=gatewayout
  Reinterpret : xbsIndex_r4/Reinterpret  force_arith_type=on  arith_type=Unsigned  force_bin_pt=on  bin_pt=0  block_type=reinterpret
  Scope : Scope  NumInputPorts=4
  Terminator : Terminator
  c_to_ri : Subsystem
  c_to_ri1 : Subsystem
  cmult_dsp48e : Subsystem  AncestorBlock=casper_library_multipliers/cmult_dsp48e
  real : Subsystem  Tag=xps:bram  AncestorBlock=xps_library/Shared_BRAM
  vacc_32bit : Subsystem
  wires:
  Gateway Out3/1 -> Scope/4
  Gateway Out2/1 -> Scope/3
  Gateway Out1/1 -> Scope/2
  Gateway Out/1 -> Scope/1
  real/1(data_out) -> Terminator/1
  cmult_dsp48e/1(c_re) -> vacc_32bit/1(din)
  new_acc/1 -> Delay3/1
  vacc_32bit/1(dout) -> Reinterpret/1
  c_to_ri/1(re) -> cmult_dsp48e/1(a_re)
  c_to_ri/2(im) -> cmult_dsp48e/2(a_im)
  c_to_ri1/1(re) -> cmult_dsp48e/3(b_re)
  c_to_ri1/2(im) -> cmult_dsp48e/4(b_im)
  a+bi/1 -> c_to_ri/1(c)
  c+di/1 -> c_to_ri1/1(c)
  Delay3/1 -> Gateway Out3/1, vacc_32bit/2(new_acc), Counter/1
  vacc_32bit/2(valid) -> Gateway Out2/1, real/3(we), Counter/2
  Counter/1 -> Gateway Out/1, real/1(addr)
  Reinterpret/1 -> Gateway Out1/1, real/2(data_in)

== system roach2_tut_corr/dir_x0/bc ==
  a+bi : Inport
  c+di : Inport  Port=2
  new_acc : Inport  Port=3
  Counter : xbsIndex_r4/Counter  cnt_type=Free Running  cnt_to=Inf  operation=Up  start_count=0  cnt_by_val=1  arith_type=Unsigned  n_bits=11  bin_pt=0  load_pin=off  rst=on  en=on  explicit_period=off  period=1  dbl_ovrd=off  use_behavioral_HDL=off  implementation=Fabric  use_rpm=on  block_type=counter
  Delay3 : xbsIndex_r4/Delay  rst=off  infoeditControl=Selection of Reset will increase slice count due to use of real FFs and instead of SRLs  en=off  latency=4  dbl_ovrd=off  reg_retiming=off  block_type=delay
  Reinterpret : xbsIndex_r4/Reinterpret  force_arith_type=on  arith_type=Unsigned  force_bin_pt=on  bin_pt=0  block_type=reinterpret
  Reinterpret1 : xbsIndex_r4/Reinterpret  force_arith_type=on  arith_type=Unsigned  force_bin_pt=on  bin_pt=0  block_type=reinterpret
  c_to_ri : Subsystem
  c_to_ri1 : Subsystem
  cmult_dsp48e : Subsystem  AncestorBlock=casper_library_multipliers/cmult_dsp48e
  imag : Subsystem  Tag=xps:bram  AncestorBlock=xps_library/Shared_BRAM
  real : Subsystem  Tag=xps:bram  AncestorBlock=xps_library/Shared_BRAM
  vacc_0 : Subsystem
  vacc_1 : Subsystem
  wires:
  Counter/1 -> real/1(addr), imag/1(addr)
  vacc_1/1(dout) -> Reinterpret1/1
  Reinterpret1/1 -> imag/2(data_in)
  vacc_1/2(valid) -> imag/3(we)
  Reinterpret/1 -> real/2(data_in)
  vacc_0/2(valid) -> real/3(we), Counter/2
  vacc_0/1(dout) -> Reinterpret/1
  new_acc/1 -> Delay3/1
  Delay3/1 -> vacc_0/2(new_acc), Counter/1, vacc_1/2(new_acc)
  c+di/1 -> c_to_ri1/1(c)
  a+bi/1 -> c_to_ri/1(c)
  c_to_ri1/2(im) -> cmult_dsp48e/4(b_im)
  c_to_ri1/1(re) -> cmult_dsp48e/3(b_re)
  c_to_ri/2(im) -> cmult_dsp48e/2(a_im)
  c_to_ri/1(re) -> cmult_dsp48e/1(a_re)
  cmult_dsp48e/2(c_im) -> vacc_1/1(din)
  cmult_dsp48e/1(c_re) -> vacc_0/1(din)

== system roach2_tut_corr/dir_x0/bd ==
  a+bi : Inport
  c+di : Inport  Port=2
  new_acc : Inport  Port=3
  Counter : xbsIndex_r4/Counter  cnt_type=Free Running  cnt_to=Inf  operation=Up  start_count=0  cnt_by_val=1  arith_type=Unsigned  n_bits=11  bin_pt=0  load_pin=off  rst=on  en=on  explicit_period=off  period=1  dbl_ovrd=off  use_behavioral_HDL=off  implementation=Fabric  use_rpm=on  block_type=counter
  Delay3 : xbsIndex_r4/Delay  rst=off  infoeditControl=Selection of Reset will increase slice count due to use of real FFs and instead of SRLs  en=off  latency=4  dbl_ovrd=off  reg_retiming=off  block_type=delay
  Reinterpret : xbsIndex_r4/Reinterpret  force_arith_type=on  arith_type=Unsigned  force_bin_pt=on  bin_pt=0  block_type=reinterpret
  Reinterpret1 : xbsIndex_r4/Reinterpret  force_arith_type=on  arith_type=Unsigned  force_bin_pt=on  bin_pt=0  block_type=reinterpret
  c_to_ri : Subsystem
  c_to_ri1 : Subsystem
  cmult_dsp48e : Subsystem  AncestorBlock=casper_library_multipliers/cmult_dsp48e
  imag : Subsystem  Tag=xps:bram  AncestorBlock=xps_library/Shared_BRAM
  real : Subsystem  Tag=xps:bram  AncestorBlock=xps_library/Shared_BRAM
  vacc_0 : Subsystem
  vacc_1 : Subsystem
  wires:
  cmult_dsp48e/1(c_re) -> vacc_0/1(din)
  cmult_dsp48e/2(c_im) -> vacc_1/1(din)
  c_to_ri/1(re) -> cmult_dsp48e/1(a_re)
  c_to_ri/2(im) -> cmult_dsp48e/2(a_im)
  c_to_ri1/1(re) -> cmult_dsp48e/3(b_re)
  c_to_ri1/2(im) -> cmult_dsp48e/4(b_im)
  a+bi/1 -> c_to_ri/1(c)
  c+di/1 -> c_to_ri1/1(c)
  Delay3/1 -> vacc_1/2(new_acc), Counter/1, vacc_0/2(new_acc)
  new_acc/1 -> Delay3/1
  vacc_0/1(dout) -> Reinterpret/1
  vacc_0/2(valid) -> Counter/2, real/3(we)
  Reinterpret/1 -> real/2(data_in)
  vacc_1/2(valid) -> imag/3(we)
  Reinterpret1/1 -> imag/2(data_in)
  vacc_1/1(dout) -> Reinterpret1/1
  Counter/1 -> imag/1(addr), real/1(addr)

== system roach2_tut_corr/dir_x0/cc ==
  a+bi : Inport
  c+di : Inport  Port=2
  new_acc : Inport  Port=3
  Counter : xbsIndex_r4/Counter  cnt_type=Free Running  cnt_to=Inf  operation=Up  start_count=0  cnt_by_val=1  arith_type=Unsigned  n_bits=chan_bits  bin_pt=0  load_pin=off  rst=on  en=on  explicit_period=off  period=1  dbl_ovrd=off  use_behavioral_HDL=off  implementation=Fabric  use_rpm=on  block_type=counter
  Delay3 : xbsIndex_r4/Delay  rst=off  infoeditControl=Selection of Reset will increase slice count due to use of real FFs and instead of SRLs  en=off  latency=4  dbl_ovrd=off  reg_retiming=off  block_type=delay
  Gateway Out{,1..3} (4 alike) : xbsIndex_r4/Gateway Out  inherit_from_input=off  hdl_port=on  timing_constraint=None  locs_specified=off  LOCs={}  UseAsDAC=off  DACChannel='1'  block_type=gatewayout
  Reinterpret : xbsIndex_r4/Reinterpret  force_arith_type=on  arith_type=Unsigned  force_bin_pt=on  bin_pt=0  block_type=reinterpret
  Scope : Scope  NumInputPorts=4
  Terminator : Terminator
  c_to_ri : Subsystem
  c_to_ri1 : Subsystem
  cmult_dsp48e : Subsystem  AncestorBlock=casper_library_multipliers/cmult_dsp48e
  real : Subsystem  Tag=xps:bram  AncestorBlock=xps_library/Shared_BRAM
  vacc_32bit : Subsystem
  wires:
  Reinterpret/1 -> real/2(data_in), Gateway Out1/1
  Counter/1 -> real/1(addr), Gateway Out/1
  vacc_32bit/2(valid) -> Counter/2, real/3(we), Gateway Out2/1
  Delay3/1 -> Counter/1, vacc_32bit/2(new_acc), Gateway Out3/1
  c+di/1 -> c_to_ri1/1(c)
  a+bi/1 -> c_to_ri/1(c)
  c_to_ri1/2(im) -> cmult_dsp48e/4(b_im)
  c_to_ri1/1(re) -> cmult_dsp48e/3(b_re)
  c_to_ri/2(im) -> cmult_dsp48e/2(a_im)
  c_to_ri/1(re) -> cmult_dsp48e/1(a_re)
  vacc_32bit/1(dout) -> Reinterpret/1
  new_acc/1 -> Delay3/1
  cmult_dsp48e/1(c_re) -> vacc_32bit/1(din)
  real/1(data_out) -> Terminator/1
  Gateway Out/1 -> Scope/1
  Gateway Out1/1 -> Scope/2
  Gateway Out2/1 -> Scope/3
  Gateway Out3/1 -> Scope/4
